TYPE APCControlAI :
STRUCT
	Value_sensor_input1_p1	:	REAL	;
	Value_sensor_input1_p2	:	REAL	;
	Select_controller_using	:	REAL	;
	Position_actual_value	:	REAL	;
	Control_mode_status	:	REAL	;
	HOME_status	:	REAL	;
	Warning_Device_Management	:	REAL	;
	Warning_Sensor_Input1	:	REAL	;
	Warning_Sensor_Input2	:	REAL	;
	Warning_Process_Controller_Selector	:	REAL	;
	Warning_Valve	:	REAL	;
	Manufacturer_Warning_Valve	:	REAL	;
	ERROR_Device_Management	:	REAL	;
	ERROR_sensor_input1_p1	:	REAL	;
	ERROR_sensor_input1_p2	:	REAL	;
	ERROR_Valve	:	REAL	;

END_STRUCT
END_TYPE
